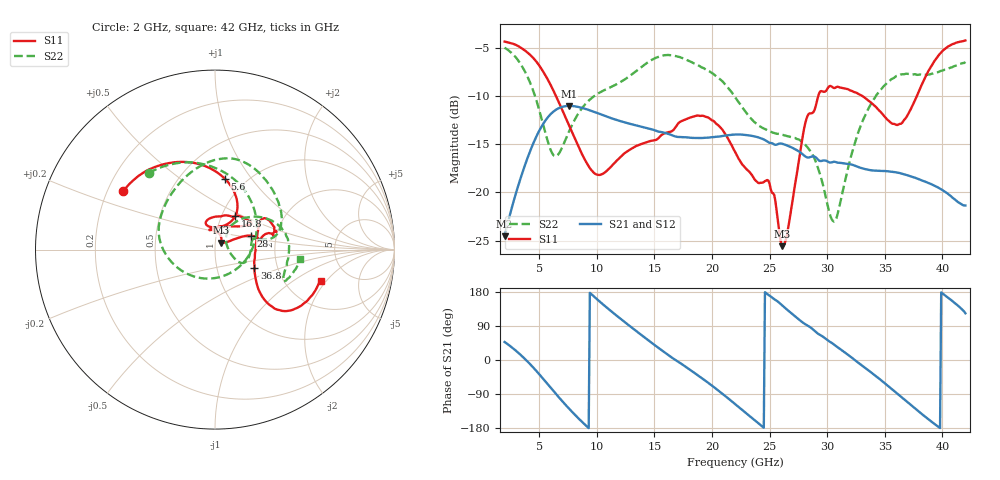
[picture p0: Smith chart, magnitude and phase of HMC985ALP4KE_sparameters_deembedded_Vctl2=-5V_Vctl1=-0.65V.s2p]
!s2p File: Measurements: S11, S21, S12, S22
# GHz S dB R 50.0
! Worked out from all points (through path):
!   401 points, 2 GHz to 42 GHz, reference 50 ohm
!   highest |S21| = -11.02 dB at 7.6 GHz (marker M1); lowest = -24.6 dB at 2 GHz (marker M2)
!   lowest |S11| = -25.6 dB at 26.1 GHz (marker M3), VSWR 1.11, Z = 53.5 + j4.16 ohm
!   |S11| at or under -10 dB: 6.461 GHz to 29.23 GHz (22.76 GHz wide, 128 % of centre); 33.07 GHz to 37.78 GHz (4.711 GHz wide, 13.3 % of centre)
!   |S22| runs from -23.0 to -5.0 dB; largest |S21 - S12| = 0.00027
!   S11 on the Smith chart (normalised r, x): 2 GHz: 0.26, +0.27; 5.6 GHz: 0.80, +0.75; 16.8 GHz: 1.16, +0.45; 28 GHz: 1.48, +0.24; 36.8 GHz: 1.52, -0.33; 42 GHz: 3.10, -1.77
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2  -4.34 147.4  -24.57 47.6  -24.57 47.6  -4.97 130.9
3.6  -5.13 120.7  -17.75 7.6  -17.75 7.6  -7.09 85.8
4.7  -6.34 99.9  -14.34 -27.0  -14.34 -26.9  -10.22 44.1
5.6  -7.97 82.3  -12.44 -58.6  -12.44 -58.6  -14.08 -5.2
6.5  -10.10 67.7  -11.38 -91.0  -11.39 -91.0  -16.22 -75.1
7.6  -13.05 58.9  -11.02 -128.6  -11.02 -128.6  -13.65 -140.5
8.7  -15.98 63.9  -11.21 -162.6  -11.22 -162.6  -11.28 -173.3
11.9  -16.51 109.4  -12.54 112.7  -12.55 112.7  -8.65 140.0
15.4  -14.31 77.5  -13.70 31.1  -13.70 31.1  -5.91 86.5
16.8  -13.30 58.9  -14.19 0.6  -14.19 0.7  -5.83 69.8
19.5  -12.16 35.2  -14.32 -56.2  -14.33 -56.2  -7.27 33.9
22  -15.77 52.7  -13.99 -116.1  -14.00 -116.1  -10.09 11.0
24.9  -18.77 100.2  -14.79 171.8  -14.79 171.8  -13.60 12.3
26.1  -25.58 47.5  -14.95 144.0  -14.96 144.0  -14.01 -0.9
28  -13.36 21.2  -16.17 96.4  -16.18 96.5  -14.92 -23.8
28.7  -11.76 11.3  -16.26 82.4  -16.27 82.5  -15.98 -27.3
30.7  -9.14 19.2  -16.83 38.2  -16.83 38.2  -22.96 24.6
32.9  -9.89 32.7  -17.45 -11.7  -17.45 -11.7  -13.12 49.9
35.4  -12.62 10.4  -17.82 -71.3  -17.82 -71.2  -8.44 21.0
36.8  -12.32 -24.8  -18.16 -106.9  -18.17 -106.9  -7.69 3.8
39.6  -5.90 -42.4  -19.47 -175.1  -19.47 -175.0  -7.52 -24.4
42  -4.22 -16.8  -21.35 123.2  -21.35 123.3  -6.45 -6.2
